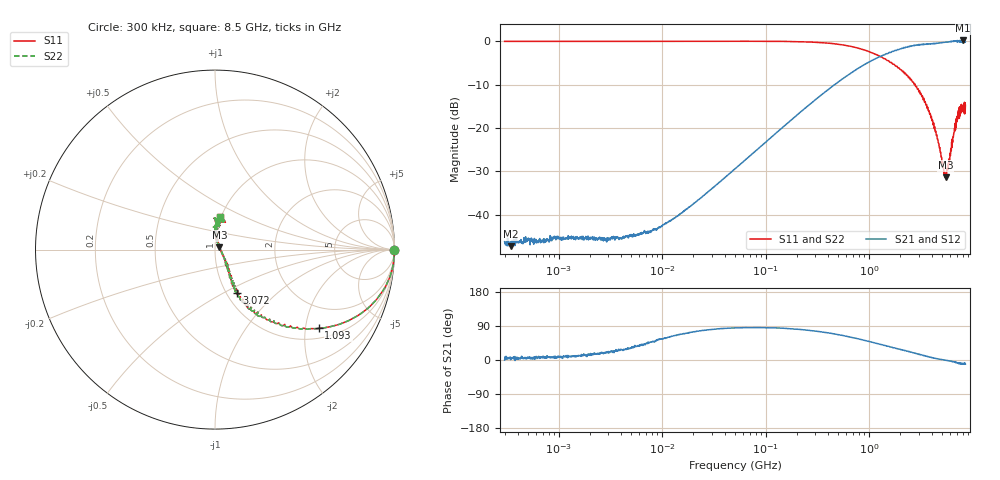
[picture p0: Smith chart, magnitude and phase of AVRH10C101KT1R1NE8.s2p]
! S-Parameter Data Generated by TDK Corporation
! Copyright(C) 2023 TDK Corporation.
! All Rights Reserved.
! TDK P/N: AVRH10C101KT1R1NE8 (Varistor)
! Property: V1mA=110V
! Size(LxWxT): 1x0.5x0.5mm
! Model Type: s2p (Touchstone File Format Version 1.0)
! Frequency: DC=Yes Start=0.3MHz Stop=8500MHz 1602points Log-sweep
! Model Generated on Oct. 12, 2023
! Port Assignments:
!  1 ---N--- 2
! Applicable Conditions:
!  Temperature = 25 degC
!  DC Bias Voltage = 0 V
!  Small Signal Operation
! Terms and conditions regarding TDK Simulation Models
! (1)This simulation model is being provided solely for informational purposes. Please refer to the specifications of the products in terms of detailed characteristics of such products.
! (2)In no event shall TDK Corporation of any of its subsidiaries be liable for any loss or damage arising, directly or indirectly,
!  From any information contained in this simulation model, including, but not limited to loss or damages arising from any inaccuracies, omissions or errors in connection with such information.
! (3)Any and all copyrights on this simulation model are owned by TDK Corporation.
!  Duplication or redistribution of this simulation model without prior written permission from TDK Corporation is prohibited.
! (4)This simulation model is subject to any modification or change without any prior notice.
! (5)Neither TDK Corporation nor any of its subsidiaries shall make any warranty, express or implied,
!  Including but not limited to the correctness, implied warranties of merchantability and fitness for a particular purpose with respect to this simulation models.
! (6)The use of this simulation model shall be deemed to have consented to the terms and conditions hereof.
# Hz S MA R 50
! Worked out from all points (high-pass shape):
!   1601 points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, 300 kHz to 8.5 GHz, reference 50 ohm
!   highest |S21| = 0.17 dB at 8.079 GHz (marker M1); lowest = -47.2 dB at 345.2 kHz (marker M2)
!   |S21| within 3 dB of the highest: 1.519 GHz to end of sweep
!   lowest |S11| = -31.4 dB at 5.491 GHz (marker M3), VSWR 1.06, Z = 52.4 + j1.27 ohm
!   |S11| at or under -10 dB: 2.778 GHz to end of sweep
!   |S22| runs from -31.4 to 0.0 dB; largest |S21 - S12| = 0
!   S11 on the Smith chart (normalised r, x): 300 kHz: open; 1.093 GHz: 1.28, -2.37; 3.072 GHz: 1.12, -0.58; 8.5 GHz: 0.99, +0.37
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300000  0.9951 0.0  0.004919 -0.3  0.004919 -0.3  0.9951 0.0
345164  0.9957 -0.0  0.004349 6.7  0.004349 6.7  0.9957 -0.0
1656733  0.9946 -0.1  0.005615 14.7  0.005615 14.7  0.9946 -0.1
3980098  0.9952 -0.1  0.005418 28.4  0.005418 28.4  0.9952 -0.1
9166247  0.9959 -0.3  0.007074 54.6  0.007074 54.6  0.9959 -0.3
1.834619e7  0.9964 -0.7  0.01229 72.6  0.01229 72.6  0.9964 -0.7
5.049752e7  0.9974 -1.9  0.03388 84.6  0.03388 84.6  0.9974 -1.9
2.806623e8  0.9757 -11.3  0.1963 77.3  0.1963 77.3  0.9757 -11.3
5.831012e8  0.8974 -22.6  0.3845 63.6  0.3845 63.6  0.8974 -22.6
1.092981e9  0.7259 -37.2  0.6087 46.1  0.6087 46.1  0.7259 -37.2
1.543407e9  0.5936 -46.7  0.7336 36.1  0.7336 36.1  0.5936 -46.7
2.243044e9  0.4266 -57.2  0.8481 25.0  0.8481 25.0  0.4266 -57.2
3.07222e9  0.2681 -63.3  0.9118 15.2  0.9118 15.2  0.2681 -63.3
4.109257e9  0.1216 -55.1  0.9357 6.1  0.9357 6.1  0.1216 -55.1
4.643188e9  0.06787 -42.1  0.9507 2.7  0.9507 2.7  0.06787 -42.1
5.219981e9  0.03517 -10.6  0.9655 0.4  0.9655 0.4  0.03517 -10.6
5.491412e9  0.02694 26.8  0.976 -0.7  0.976 -0.7  0.02694 26.8
5.830702e9  0.03949 58.6  0.98 -2.0  0.98 -2.0  0.03949 58.6
7.004263e9  0.1168 82.4  0.9913 -6.7  0.9913 -6.7  0.1168 82.4
7.424939e9  0.129 79.2  0.9841 -7.4  0.9841 -7.4  0.129 79.2
8.079324e9  0.1732 91.4  1.019 -9.8  1.019 -9.8  0.1732 91.4
8.5e9  0.1822 81.0  0.9879 -10.5  0.9879 -10.5  0.1822 81.0
